FUNCTION "FC_GRP_44" : VOID
TITLE =GROUP =44
{ S7_language := '9(1) Angielski (Stany Zjednoczone)  11.01.2022  09:45:15' }
VERSION : 0.1


VAR_TEMP
  CL : "UDT_CABINET";	//CABINET LOCAL
  CR : "UDT_CABINET";	//CABINET REMOTE
  RelError : BOOL ;	//ERROR RELEASE
  RelErrorCL : BOOL ;	//ERROR RELEASE FROM CABINET LOCAL
  RelErrorCR : BOOL ;	//ERROR RELEASE FROM CABINET REMOTE
  RelControl : BOOL ;	//CONTROL RELEASE
  RelControlCL : BOOL ;	//CONTROL RELEASE FROM CABINET LOCAL
  RelControlCR : BOOL ;	//CONTROL RELEASE FROM CABINET REMOTE
  ErrorConfirm : BOOL ;	//ERROR CONFIRM
  AutoOn : BOOL ;	//AUTOMATIC ON
  AutoOff : BOOL ;	//AUTOMATIC OFF
  RelAuto : BOOL ;	//AUTOMATIC RELEASE
  TempSetpoint : REAL ;
  LAMP_ON : BOOL ;
END_VAR
BEGIN
NETWORK
TITLE =GLOBAL SIGNALS
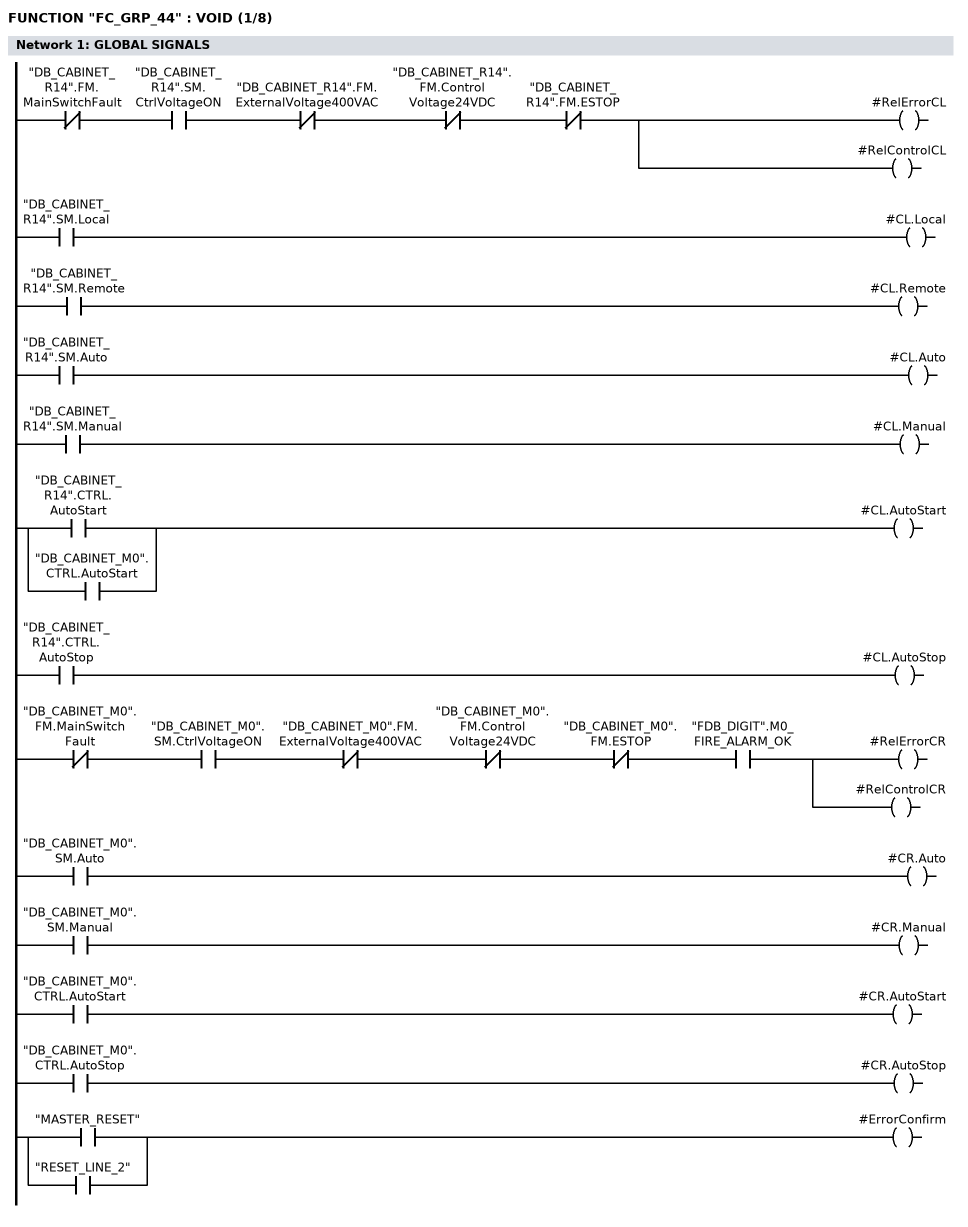
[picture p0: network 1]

//LOCAL
      UN    "DB_CABINET_R14".FM.MainSwitchFault;
      U     "DB_CABINET_R14".SM.CtrlVoltageON;
      UN    "DB_CABINET_R14".FM.ExternalVoltage400VAC;
      UN    "DB_CABINET_R14".FM.ControlVoltage24VDC;
      UN    "DB_CABINET_R14".FM.ESTOP;
      =     #RelErrorCL;
      =     #RelControlCL;

      U     "DB_CABINET_R14".SM.Local;
      =     #CL.Local;
      U     "DB_CABINET_R14".SM.Remote;
      =     #CL.Remote;
      U     "DB_CABINET_R14".SM.Auto;
      =     #CL.Auto;
      U     "DB_CABINET_R14".SM.Manual;
      =     #CL.Manual;
      U     "DB_CABINET_R14".CTRL.AutoStart;
      O     "DB_CABINET_M0".CTRL.AutoStart;
      =     #CL.AutoStart;
      U     "DB_CABINET_R14".CTRL.AutoStop;
      =     #CL.AutoStop;


//REMOTE

      UN    "DB_CABINET_M0".FM.MainSwitchFault;
      U     "DB_CABINET_M0".SM.CtrlVoltageON;
      UN    "DB_CABINET_M0".FM.ExternalVoltage400VAC;
      UN    "DB_CABINET_M0".FM.ControlVoltage24VDC;
//      UN    "DB_CABINET_M0".FM.ControlVoltage230VAC_MS
      UN    "DB_CABINET_M0".FM.ESTOP;
      U     "FDB_DIGIT".M0_FIRE_ALARM_OK;
      =     #RelErrorCR;
      =     #RelControlCR;

      U     "DB_CABINET_M0".SM.Auto;
      =     #CR.Auto;
      U     "DB_CABINET_M0".SM.Manual;
      =     #CR.Manual;
      U     "DB_CABINET_M0".CTRL.AutoStart;
      =     #CR.AutoStart;
      U     "DB_CABINET_M0".CTRL.AutoStop;
      =     #CR.AutoStop;

      U     "MASTER_RESET";
      O     "RESET_LINE_2";
      =     #ErrorConfirm;

NETWORK
TITLE =GLOBAL SIGNALS - GROUP GENERAL ERROR AND WARNING
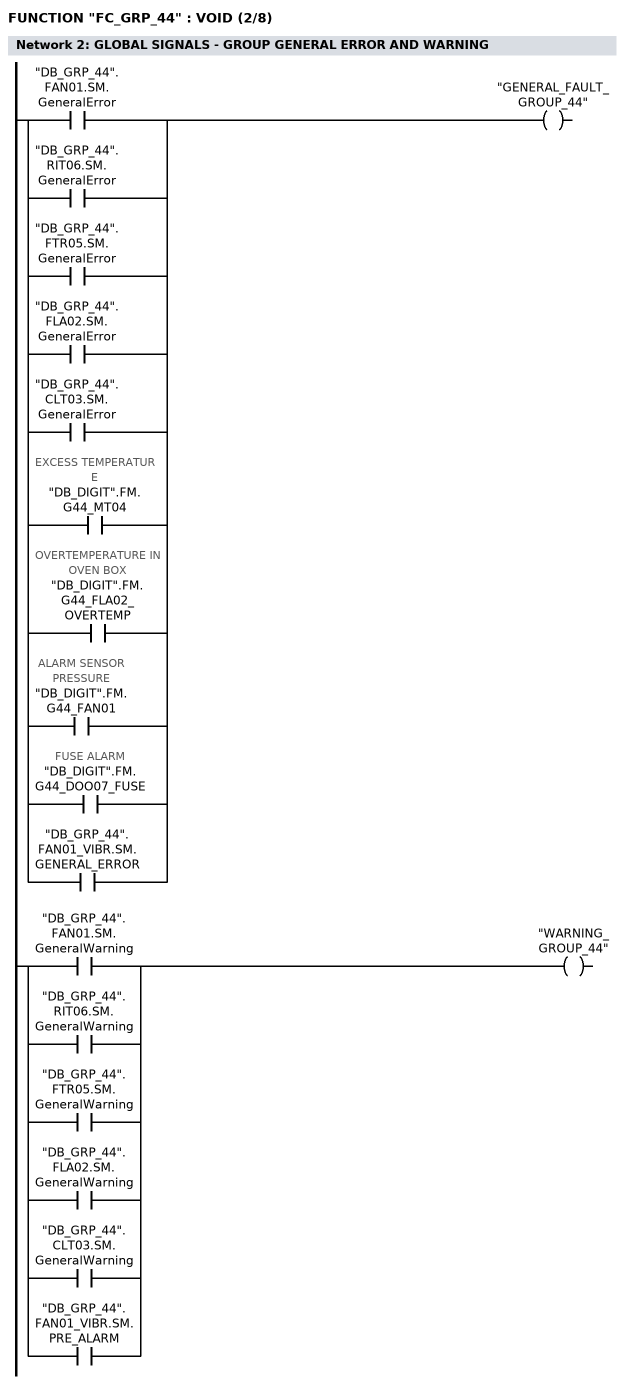
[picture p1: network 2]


      U     "DB_GRP_44".FAN01.SM.GeneralError;
      O     "DB_GRP_44".RIT06.SM.GeneralError;
      O     "DB_GRP_44".FTR05.SM.GeneralError;
      O     "DB_GRP_44".FLA02.SM.GeneralError;
      O     "DB_GRP_44".CLT03.SM.GeneralError;
      O     "DB_DIGIT".FM.G44_MT04; //EXCESS TEMPERATURE
      O     "DB_DIGIT".FM.G44_FLA02_OVERTEMP; //OVERTEMPERATURE IN OVEN BOX
      O     "DB_DIGIT".FM.G44_FAN01; //ALARM SENSOR PRESSURE
      O     "DB_DIGIT".FM.G44_DOO07_FUSE; //FUSE ALARM
      O     "DB_GRP_44".FAN01_VIBR.SM.GENERAL_ERROR;
      =     "GENERAL_FAULT_GROUP_44";

      U     "DB_GRP_44".FAN01.SM.GeneralWarning;
      O     "DB_GRP_44".RIT06.SM.GeneralWarning;
      O     "DB_GRP_44".FTR05.SM.GeneralWarning;
      O     "DB_GRP_44".FLA02.SM.GeneralWarning;
      O     "DB_GRP_44".CLT03.SM.GeneralWarning;
      O     "DB_GRP_44".FAN01_VIBR.SM.PRE_ALARM;
      =     "WARNING_GROUP_44";


NETWORK
TITLE =RELEASE CONTROL
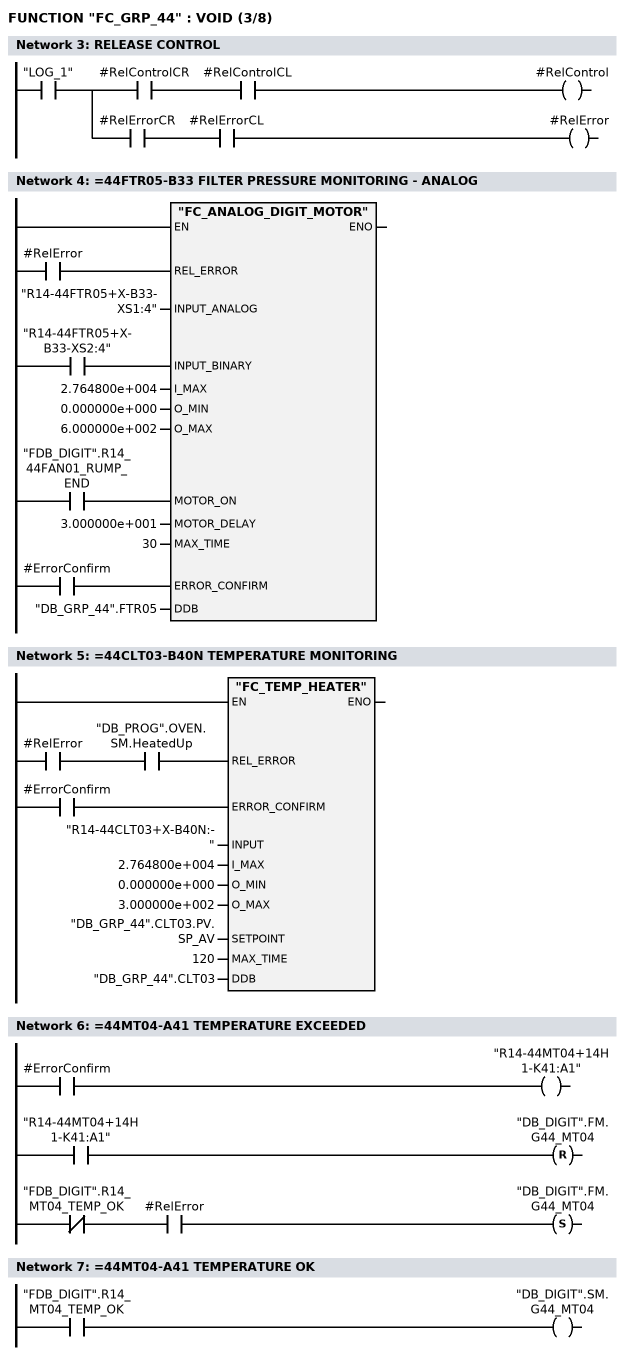
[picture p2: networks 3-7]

      U     "LOG_1";
      =     L     11.0;
      U     L     11.0;
      U     #RelControlCR;
      U     #RelControlCL;
      =     #RelControl;
      U     L     11.0;
      U     #RelErrorCR;
      U     #RelErrorCL;
      =     #RelError;
NETWORK
TITLE ==44FTR05-B33 FILTER PRESSURE MONITORING - ANALOG

      U     #RelError;
      =     L     11.0;
      BLD   103;
      U     "R14-44FTR05+X-B33-XS2:4";
      =     L     11.1;
      BLD   103;
      U     "FDB_DIGIT".R14_44FAN01_RUMP_END;
      =     L     11.2;
      BLD   103;
      U     #ErrorConfirm;
      =     L     11.3;
      BLD   103;
      CALL "FC_ANALOG_DIGIT_MOTOR" (
           REL_ERROR                := L     11.0,
           INPUT_ANALOG             := "R14-44FTR05+X-B33-XS1:4",
           INPUT_BINARY             := L     11.1,
           I_MAX                    := 2.764800e+004,
           O_MIN                    := 0.000000e+000,
           O_MAX                    := 6.000000e+002,
           MOTOR_ON                 := L     11.2,
           MOTOR_DELAY              := 3.000000e+001,
           MAX_TIME                 := 30,
           ERROR_CONFIRM            := L     11.3,
           DDB                      := "DB_GRP_44".FTR05);
      NOP   0;
NETWORK
TITLE ==44CLT03-B40N TEMPERATURE MONITORING

      U     #RelError;
      U     "DB_PROG".OVEN.SM.HeatedUp;
      =     L     11.0;
      BLD   103;
      U     #ErrorConfirm;
      =     L     11.1;
      BLD   103;
      CALL "FC_TEMP_HEATER" (
           REL_ERROR                := L     11.0,
           ERROR_CONFIRM            := L     11.1,
           INPUT                    := "R14-44CLT03+X-B40N:-",
           I_MAX                    := 2.764800e+004,
           O_MIN                    := 0.000000e+000,
           O_MAX                    := 3.000000e+002,
           SETPOINT                 := "DB_GRP_44".CLT03.PV.SP_AV,
           MAX_TIME                 := 120,
           DDB                      := "DB_GRP_44".CLT03);
      NOP   0;
NETWORK
TITLE ==44MT04-A41 TEMPERATURE EXCEEDED

      U     #ErrorConfirm;
      =     "R14-44MT04+14H1-K41:A1";
      U     "R14-44MT04+14H1-K41:A1";
      R     "DB_DIGIT".FM.G44_MT04;
      UN    "FDB_DIGIT".R14_MT04_TEMP_OK;
      U     #RelError;
      S     "DB_DIGIT".FM.G44_MT04;
      NOP   0;
NETWORK
TITLE ==44MT04-A41 TEMPERATURE OK

      U     "FDB_DIGIT".R14_MT04_TEMP_OK;
      =     "DB_DIGIT".SM.G44_MT04;
NETWORK
TITLE ==44DOO07-F1.1 ACCESS DOOR FUSE ERROR
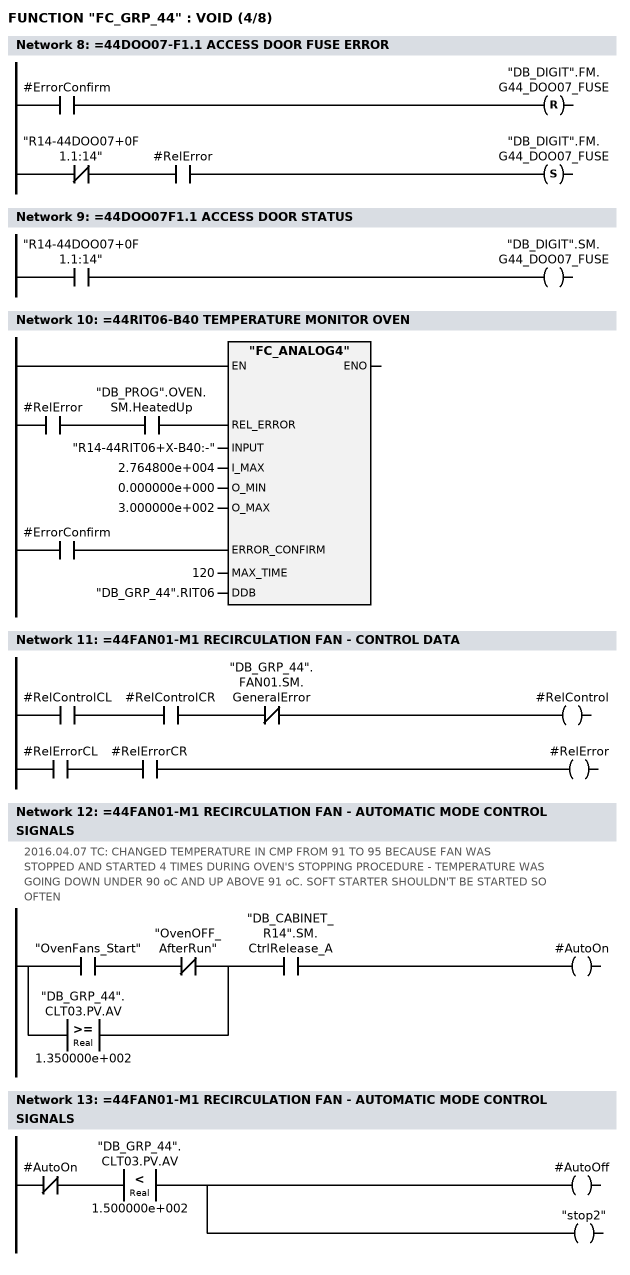
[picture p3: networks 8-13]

      U     #ErrorConfirm;
      R     "DB_DIGIT".FM.G44_DOO07_FUSE;
      UN    "R14-44DOO07+0F1.1:14";
      U     #RelError;
      S     "DB_DIGIT".FM.G44_DOO07_FUSE;
      NOP   0;
NETWORK
TITLE ==44DOO07F1.1 ACCESS DOOR STATUS

      U     "R14-44DOO07+0F1.1:14";
      =     "DB_DIGIT".SM.G44_DOO07_FUSE;
NETWORK
TITLE ==44RIT06-B40 TEMPERATURE MONITOR OVEN

      U     #RelError;
      U     "DB_PROG".OVEN.SM.HeatedUp;
      =     L     11.0;
      BLD   103;
      U     #ErrorConfirm;
      =     L     11.1;
      BLD   103;
      CALL "FC_ANALOG4" (
           REL_ERROR                := L     11.0,
           INPUT                    := "R14-44RIT06+X-B40:-",
           I_MAX                    := 2.764800e+004,
           O_MIN                    := 0.000000e+000,
           O_MAX                    := 3.000000e+002,
           ERROR_CONFIRM            := L     11.1,
           MAX_TIME                 := 120,
           DDB                      := "DB_GRP_44".RIT06);
      NOP   0;
NETWORK
TITLE ==44FAN01-M1 RECIRCULATION FAN - CONTROL DATA


      U     #RelControlCL;
      U     #RelControlCR;
      UN    "DB_GRP_44".FAN01.SM.GeneralError;
      =     #RelControl;



      U     #RelErrorCL;
      U     #RelErrorCR;
      =     #RelError;
NETWORK
TITLE ==44FAN01-M1 RECIRCULATION FAN - AUTOMATIC MODE CONTROL SIGNALS
//2016.04.07 TC: CHANGED TEMPERATURE IN CMP FROM 91 TO 95 BECAUSE FAN WAS
//STOPPED AND STARTED 4 TIMES DURING OVEN'S STOPPING PROCEDURE - TEMPERATURE WAS
//GOING DOWN UNDER 90 oC AND UP ABOVE 91 oC. SOFT STARTER SHOULDN'T BE STARTED SO
//OFTEN
      U(    ;
      U     "OvenFans_Start";
      UN    "OvenOFF_AfterRun";
      O(    ;
      L     "DB_GRP_44".CLT03.PV.AV;
      L     1.350000e+002;
      >=R   ;
      )     ;
      )     ;
      U     "DB_CABINET_R14".SM.CtrlRelease_A;
      =     #AutoOn;
NETWORK
TITLE ==44FAN01-M1 RECIRCULATION FAN - AUTOMATIC MODE CONTROL SIGNALS

      UN    #AutoOn;
      U(    ;
      L     "DB_GRP_44".CLT03.PV.AV;
      L     1.500000e+002;
      <R    ;
      )     ;
      =     #AutoOff;
      =     "stop2";
NETWORK
TITLE ==44FAN01-M1 RECIRCULATION FAN
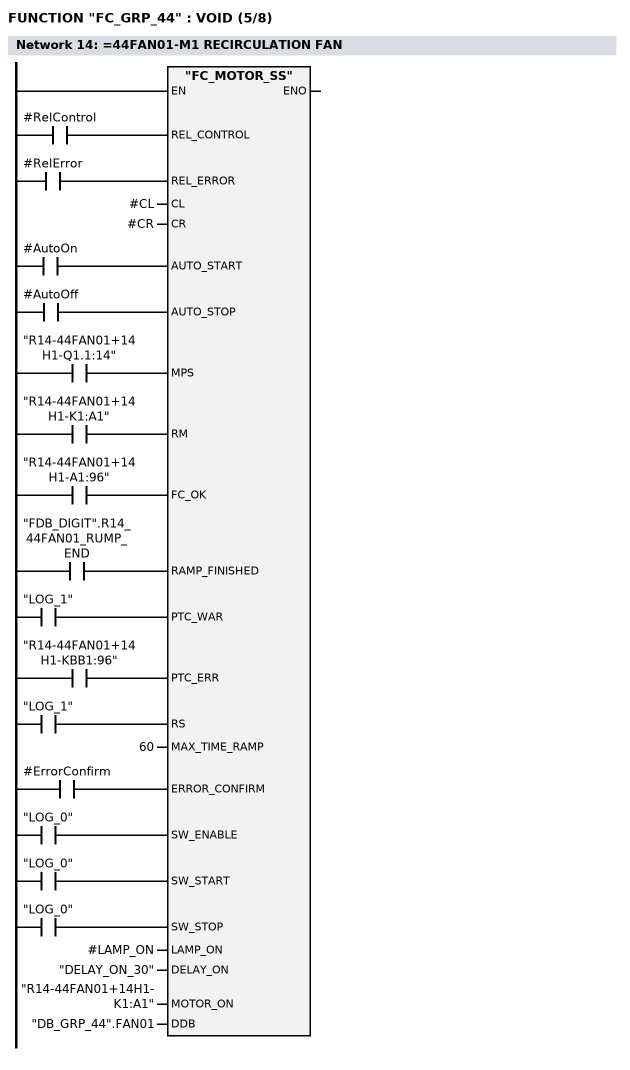
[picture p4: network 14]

      U     #RelControl;
      =     L     11.0;
      BLD   103;
      U     #RelError;
      =     L     11.1;
      BLD   103;
      U     #AutoOn;
      =     L     11.2;
      BLD   103;
      U     #AutoOff;
      =     L     11.3;
      BLD   103;
      U     "R14-44FAN01+14H1-Q1.1:14";
      =     L     11.4;
      BLD   103;
      U     "R14-44FAN01+14H1-K1:A1";
      =     L     11.5;
      BLD   103;
      U     "R14-44FAN01+14H1-A1:96";
      =     L     11.6;
      BLD   103;
      U     "FDB_DIGIT".R14_44FAN01_RUMP_END;
      =     L     11.7;
      BLD   103;
      U     "LOG_1";
      =     L     12.0;
      BLD   103;
      U     "R14-44FAN01+14H1-KBB1:96";
      =     L     12.1;
      BLD   103;
      U     "LOG_1";
      =     L     12.2;
      BLD   103;
      U     #ErrorConfirm;
      =     L     12.3;
      BLD   103;
      U     "LOG_0";
      =     L     12.4;
      BLD   103;
      U     "LOG_0";
      =     L     12.5;
      BLD   103;
      U     "LOG_0";
      =     L     12.6;
      BLD   103;
      CALL "FC_MOTOR_SS" (
           REL_CONTROL              := L     11.0,
           REL_ERROR                := L     11.1,
           CL                       := #CL,
           CR                       := #CR,
           AUTO_START               := L     11.2,
           AUTO_STOP                := L     11.3,
           MPS                      := L     11.4,
           RM                       := L     11.5,
           FC_OK                    := L     11.6,
           RAMP_FINISHED            := L     11.7,
           PTC_WAR                  := L     12.0,
           PTC_ERR                  := L     12.1,
           RS                       := L     12.2,
           MAX_TIME_RAMP            := 60,
           ERROR_CONFIRM            := L     12.3,
           SW_ENABLE                := L     12.4,
           SW_START                 := L     12.5,
           SW_STOP                  := L     12.6,
           LAMP_ON                  := #LAMP_ON,
           DELAY_ON                 := "DELAY_ON_30",
           MOTOR_ON                 := "R14-44FAN01+14H1-K1:A1",
           DDB                      := "DB_GRP_44".FAN01);
      NOP   0;
NETWORK
TITLE ==44FAN01-S32F RECIRCULATION FAN PRESSURE OK
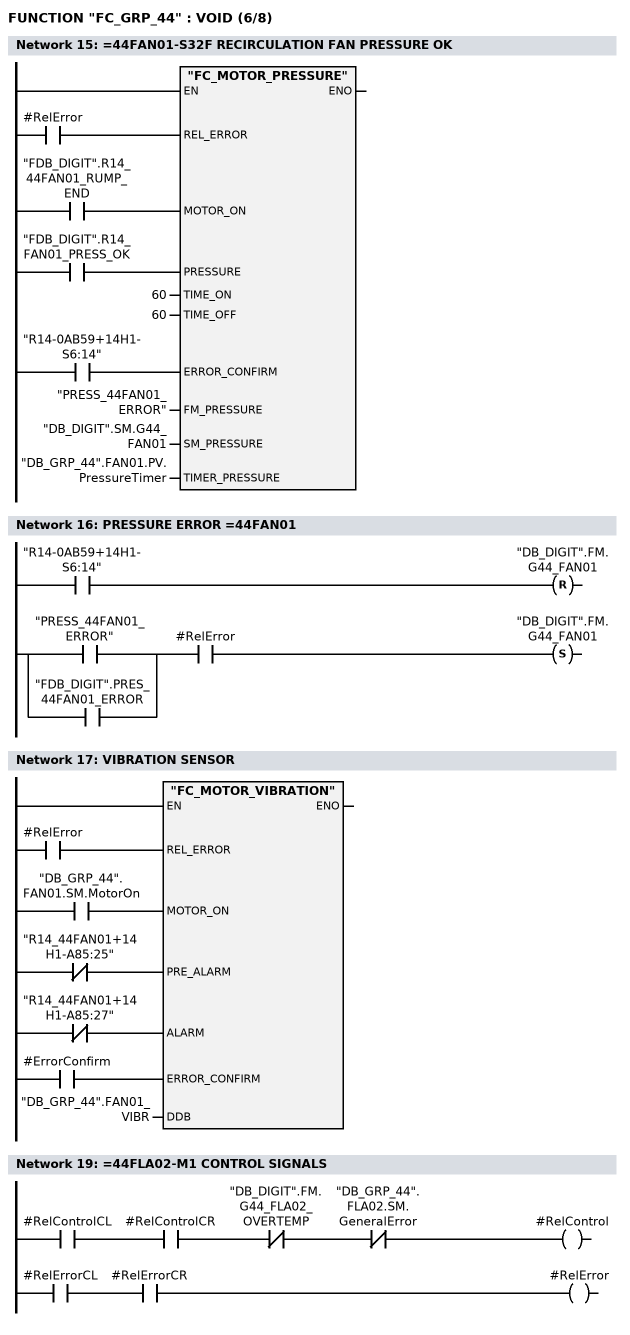
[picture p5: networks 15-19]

      U     #RelError;
      =     L     11.0;
      BLD   103;
      U     "FDB_DIGIT".R14_44FAN01_RUMP_END;
      =     L     11.1;
      BLD   103;
      U     "FDB_DIGIT".R14_FAN01_PRESS_OK;
      =     L     11.2;
      BLD   103;
      U     "R14-0AB59+14H1-S6:14";
      =     L     11.3;
      BLD   103;
      CALL "FC_MOTOR_PRESSURE" (
           REL_ERROR                := L     11.0,
           MOTOR_ON                 := L     11.1,
           PRESSURE                 := L     11.2,
           TIME_ON                  := 60,
           TIME_OFF                 := 60,
           ERROR_CONFIRM            := L     11.3,
           FM_PRESSURE              := "PRESS_44FAN01_ERROR",
           SM_PRESSURE              := "DB_DIGIT".SM.G44_FAN01,
           TIMER_PRESSURE           := "DB_GRP_44".FAN01.PV.PressureTimer);
      NOP   0;
NETWORK
TITLE =PRESSURE ERROR =44FAN01

      U     "R14-0AB59+14H1-S6:14";
      R     "DB_DIGIT".FM.G44_FAN01;
      U(    ;
      O     "PRESS_44FAN01_ERROR";
      O     "FDB_DIGIT".PRES_44FAN01_ERROR;
      )     ;
      U     #RelError;
      S     "DB_DIGIT".FM.G44_FAN01;
      NOP   0;
NETWORK
TITLE =VIBRATION SENSOR

      U     #RelError;
      =     L     11.0;
      BLD   103;
      U     "DB_GRP_44".FAN01.SM.MotorOn;
      =     L     11.1;
      BLD   103;
      UN    "R14_44FAN01+14H1-A85:25";
      =     L     11.2;
      BLD   103;
      UN    "R14_44FAN01+14H1-A85:27";
      =     L     11.3;
      BLD   103;
      U     #ErrorConfirm;
      =     L     11.4;
      BLD   103;
      CALL "FC_MOTOR_VIBRATION" (
           REL_ERROR                := L     11.0,
           MOTOR_ON                 := L     11.1,
           PRE_ALARM                := L     11.2,
           ALARM                    := L     11.3,
           ERROR_CONFIRM            := L     11.4,
           DDB                      := "DB_GRP_44".FAN01_VIBR);
      NOP   0;
NETWORK
TITLE =*********** 44FLA02 ***************

NETWORK
TITLE ==44FLA02-M1 CONTROL SIGNALS

      U     #RelControlCL;
      U     #RelControlCR;
      UN    "DB_DIGIT".FM.G44_FLA02_OVERTEMP;
      UN    "DB_GRP_44".FLA02.SM.GeneralError;
      =     #RelControl;


      U     #RelErrorCL;
      U     #RelErrorCR;
      =     #RelError;


NETWORK
TITLE ==44FLA02, CONTROL SIGNALS - AUTO_ON
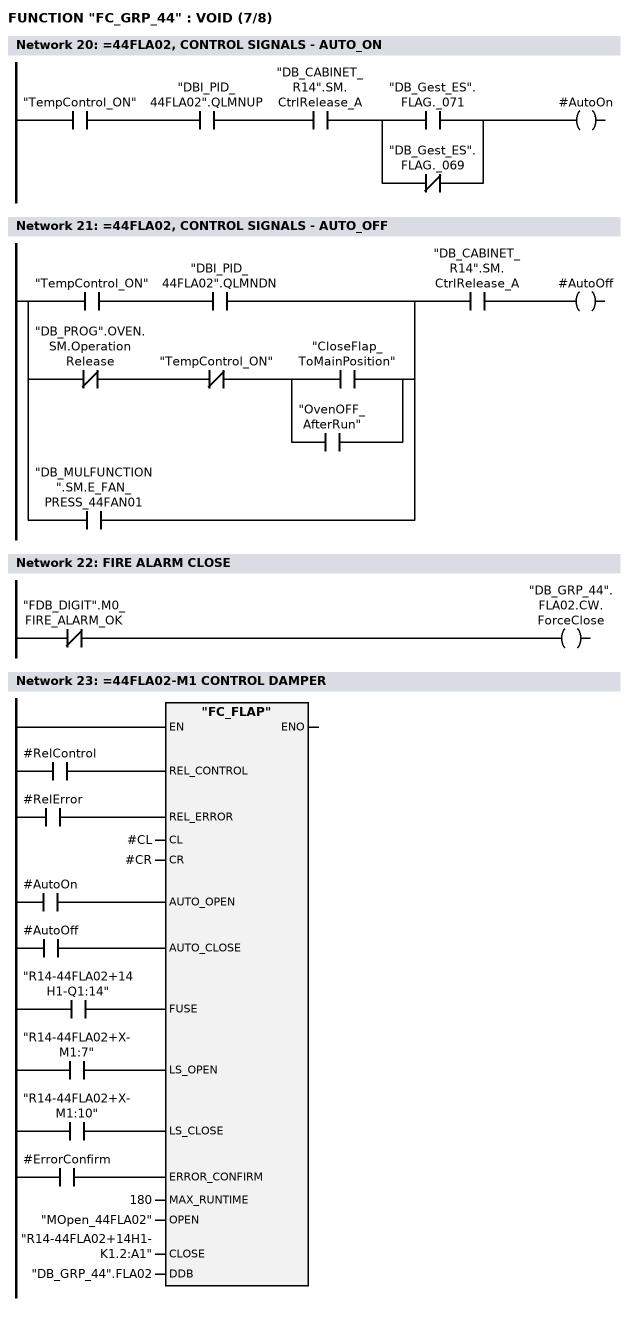
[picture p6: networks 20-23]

      U     "TempControl_ON";
      U     "DBI_PID_44FLA02".QLMNUP;
      U     "DB_CABINET_R14".SM.CtrlRelease_A;
      U(    ;
      O     "DB_Gest_ES".FLAG._071;
      ON    "DB_Gest_ES".FLAG._069;
      )     ;
      =     #AutoOn;
NETWORK
TITLE ==44FLA02, CONTROL SIGNALS - AUTO_OFF

      U(    ;
      U     "TempControl_ON";
      U     "DBI_PID_44FLA02".QLMNDN;
      O     ;
      UN    "DB_PROG".OVEN.SM.OperationRelease;
      UN    "TempControl_ON";
      U(    ;
      O     "CloseFlap_ToMainPosition";
      O     "OvenOFF_AfterRun";
      )     ;
      O     "DB_MULFUNCTION".SM.E_FAN_PRESS_44FAN01;
      )     ;
      U     "DB_CABINET_R14".SM.CtrlRelease_A;
      =     #AutoOff;
NETWORK
TITLE =FIRE ALARM CLOSE

      UN    "FDB_DIGIT".M0_FIRE_ALARM_OK;
      =     "DB_GRP_44".FLA02.CW.ForceClose;
NETWORK
TITLE ==44FLA02-M1 CONTROL DAMPER



      U     #RelControl;
      =     L     11.0;
      BLD   103;
      U     #RelError;
      =     L     11.1;
      BLD   103;
      U     #AutoOn;
      =     L     11.2;
      BLD   103;
      U     #AutoOff;
      =     L     11.3;
      BLD   103;
      U     "R14-44FLA02+14H1-Q1:14";
      =     L     11.4;
      BLD   103;
      U     "R14-44FLA02+X-M1:7";
      =     L     11.5;
      BLD   103;
      U     "R14-44FLA02+X-M1:10";
      =     L     11.6;
      BLD   103;
      U     #ErrorConfirm;
      =     L     11.7;
      BLD   103;
      CALL "FC_FLAP" (
           REL_CONTROL              := L     11.0,
           REL_ERROR                := L     11.1,
           CL                       := #CL,
           CR                       := #CR,
           AUTO_OPEN                := L     11.2,
           AUTO_CLOSE               := L     11.3,
           FUSE                     := L     11.4,
           LS_OPEN                  := L     11.5,
           LS_CLOSE                 := L     11.6,
           ERROR_CONFIRM            := L     11.7,
           MAX_RUNTIME              := 180,
           OPEN                     := "MOpen_44FLA02",
           CLOSE                    := "R14-44FLA02+14H1-K1.2:A1",
           DDB                      := "DB_GRP_44".FLA02);
      NOP   0;
NETWORK
TITLE =MANUAL INTERLOCKS - OPEN 44FLA02
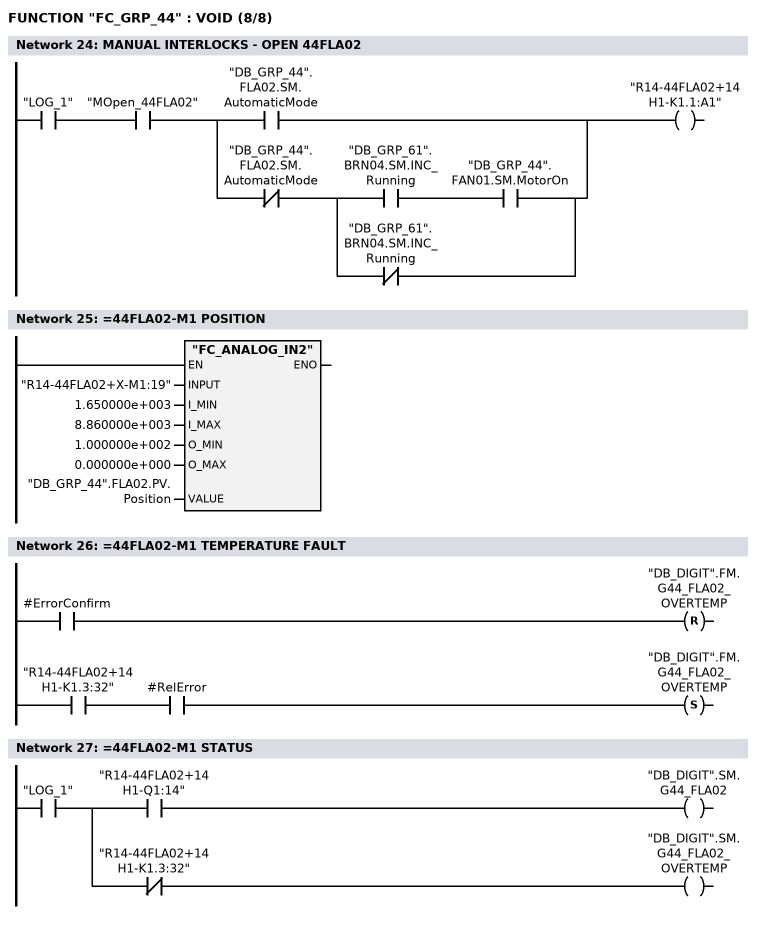
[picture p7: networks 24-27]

      U     "LOG_1";
      U     "MOpen_44FLA02";
      U(    ;
      O     "DB_GRP_44".FLA02.SM.AutomaticMode;
      O     ;
      UN    "DB_GRP_44".FLA02.SM.AutomaticMode;
      U(    ;
      U     "DB_GRP_61".BRN04.SM.INC_Running;
      U     "DB_GRP_44".FAN01.SM.MotorOn;
      ON    "DB_GRP_61".BRN04.SM.INC_Running;
      )     ;
      )     ;
      =     "R14-44FLA02+14H1-K1.1:A1";
NETWORK
TITLE ==44FLA02-M1 POSITION

      CALL "FC_ANALOG_IN2" (
           INPUT                    := "R14-44FLA02+X-M1:19",
           I_MIN                    := 1.650000e+003,
           I_MAX                    := 8.860000e+003,
           O_MIN                    := 1.000000e+002,
           O_MAX                    := 0.000000e+000,
           VALUE                    := "DB_GRP_44".FLA02.PV.Position);
      NOP   0;
NETWORK
TITLE ==44FLA02-M1 TEMPERATURE FAULT

      U     #ErrorConfirm;
      R     "DB_DIGIT".FM.G44_FLA02_OVERTEMP;
      U     "R14-44FLA02+14H1-K1.3:32";
      U     #RelError;
      S     "DB_DIGIT".FM.G44_FLA02_OVERTEMP;
      NOP   0;
NETWORK
TITLE ==44FLA02-M1 STATUS

      U     "LOG_1";
      =     L     11.0;
      U     L     11.0;
      U     "R14-44FLA02+14H1-Q1:14";
      =     "DB_DIGIT".SM.G44_FLA02;
      U     L     11.0;
      UN    "R14-44FLA02+14H1-K1.3:32";
      =     "DB_DIGIT".SM.G44_FLA02_OVERTEMP;
NETWORK
TITLE =END

END_FUNCTION

